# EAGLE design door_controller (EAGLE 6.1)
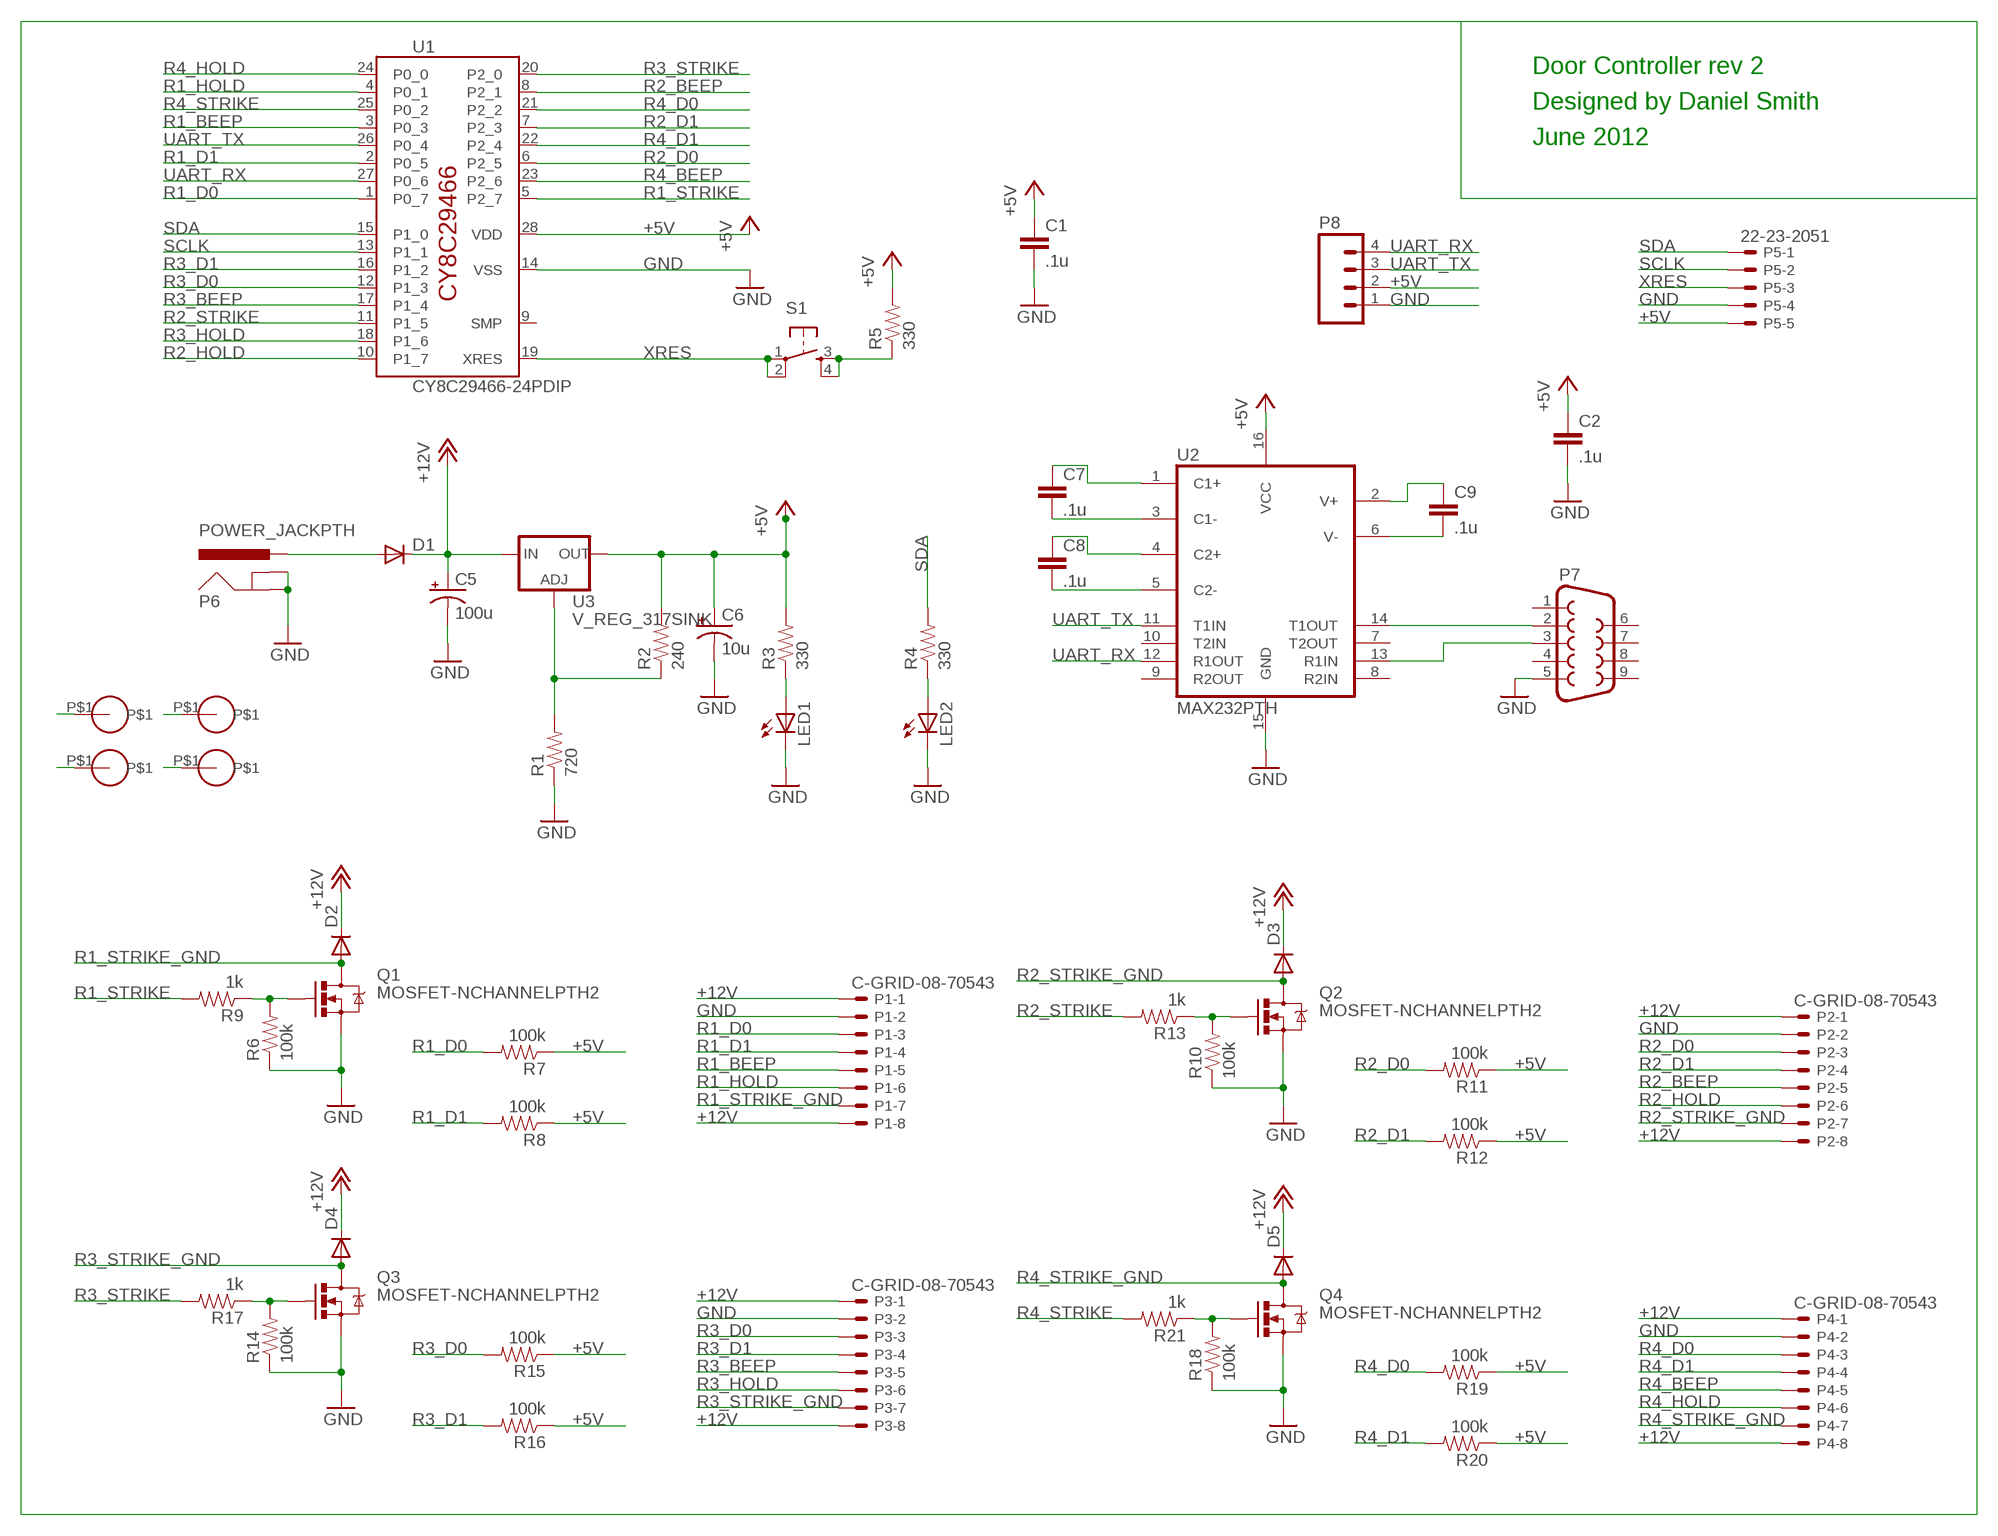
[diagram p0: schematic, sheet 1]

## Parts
C1  .1u  CAPPTH1  [CAP-PTH-5MM]
C2  .1u  CAPPTH1  [CAP-PTH-5MM]
C5  100u  CAP_POLPTH1  [CPOL-RADIAL-100UF-25V]
C6  10u  CAP_POLPTH2  [CPOL-RADIAL-10UF-25V]
C7  .1u  CAPPTH1  [CAP-PTH-5MM]
C8  .1u  CAPPTH1  [CAP-PTH-5MM]
C9  .1u  CAPPTH1  [CAP-PTH-5MM]
D1  DIODE1N4148  [DIODE-1N4148]
D2  DIODEPTH  [DIODE-1N4001]
D3  DIODEPTH  [DIODE-1N4001]
D4  DIODEPTH  [DIODE-1N4001]
D5  DIODEPTH  [DIODE-1N4001]
LED1  LED3MM  [LED3MM]
LED2  LED3MM  [LED3MM]
P1  C-GRID-08-70543  [70543-08]
P2  C-GRID-08-70543  [70543-08]
P3  C-GRID-08-70543  [70543-08]
P4  C-GRID-08-70543  [70543-08]
P5  22-23-2051  [22-23-2051]
P6  POWER_JACKPTH  [POWER_JACK_PTH]
P7  DB9FEMALE  [DB9]
P8  M04LONGPADS  [1X04_LONGPADS]
Q1  MOSFET-NCHANNELPTH2  [TO220V]
Q2  MOSFET-NCHANNELPTH2  [TO220V]
Q3  MOSFET-NCHANNELPTH2  [TO220V]
Q4  MOSFET-NCHANNELPTH2  [TO220V]
R1  720  RESISTORAXIAL-0.3  [AXIAL-0.3]
R2  240  RESISTORAXIAL-0.3  [AXIAL-0.3]
R3  330  RESISTORAXIAL-0.3  [AXIAL-0.3]
R4  330  RESISTORAXIAL-0.3  [AXIAL-0.3]
R5  330  RESISTORAXIAL-0.3  [AXIAL-0.3]
R6  100k  RESISTORAXIAL-0.3  [AXIAL-0.3]
R7  100k  RESISTORAXIAL-0.3  [AXIAL-0.3]
R8  100k  RESISTORAXIAL-0.3  [AXIAL-0.3]
R9  1k  RESISTORAXIAL-0.3  [AXIAL-0.3]
R10  100k  RESISTORAXIAL-0.3  [AXIAL-0.3]
R11  100k  RESISTORAXIAL-0.3  [AXIAL-0.3]
R12  100k  RESISTORAXIAL-0.3  [AXIAL-0.3]
R13  1k  RESISTORAXIAL-0.3  [AXIAL-0.3]
R14  100k  RESISTORAXIAL-0.3  [AXIAL-0.3]
R15  100k  RESISTORAXIAL-0.3  [AXIAL-0.3]
R16  100k  RESISTORAXIAL-0.3  [AXIAL-0.3]
R17  1k  RESISTORAXIAL-0.3  [AXIAL-0.3]
R18  100k  RESISTORAXIAL-0.3  [AXIAL-0.3]
R19  100k  RESISTORAXIAL-0.3  [AXIAL-0.3]
R20  100k  RESISTORAXIAL-0.3  [AXIAL-0.3]
R21  1k  RESISTORAXIAL-0.3  [AXIAL-0.3]
S1  TAC_SWITCHPTH  [TACTILE-PTH]
U1  CY8C29466-24PDIP  [PDIP28]
U2  MAX232PTH  [DIL16]
U3  V_REG_317SINK  [TO220-ADJ]
U$1  GNDHOLE  [GNDHOLE]
U$2  GNDHOLE  [GNDHOLE]
U$3  GNDHOLE  [GNDHOLE]
U$4  GNDHOLE  [GNDHOLE]

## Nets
+5V: C1.1 C2.1 C6.1(+) P5.5 P8.2 R2.P$2 R3.P$2 R5.P$2 R7.P$1 R8.P$1 R11.P$1 R12.P$1 R15.P$1 R16.P$1 R19.P$1 R20.P$1 U1.28(VDD) U2.16(VCC) U3.OUT
+12V [power]: C5.1(+) D1.C D2.C D3.C D4.C D5.C P1.1 P1.8 P2.1 P2.8 P3.1 P3.8 P4.1 P4.8 U3.IN
GND: C1.2 C2.2 C5.2(-) C6.2(-) LED1.K(C) LED2.K(C) P1.2 P2.2 P3.2 P4.2 P5.4 P6.GND P6.GNDBREAK P7.5 P8.1 Q1.3(S) Q2.3(S) Q3.3(S) Q4.3(S) R1.P$1 R6.P$1 R10.P$1 R14.P$1 R18.P$1 U1.14(VSS) U2.15(GND)
N$1: C7.1 U2.1(C1+)
N$2: C7.2 U2.3(C1-)
N$3: C8.1 U2.4(C2+)
N$4: C8.2 U2.5(C2-)
N$5: C9.1 U2.2(V+)
N$6: C9.2 U2.6(V-)
N$7: P7.2 U2.14(T1OUT)
N$8: P7.3 U2.13(R1IN)
N$9: U$4.P$1
N$10: R1.P$2 R2.P$1 U3.ADJ
N$11: R5.P$1 S1.3 S1.4
N$12: LED1.A R3.P$1
N$13: U$3.P$1
N$14: Q1.1(G) R6.P$2 R9.P$1
N$15: Q2.1(G) R10.P$2 R13.P$1
N$16: Q3.1(G) R14.P$2 R17.P$1
N$17: Q4.1(G) R18.P$2 R21.P$1
N$18: U$2.P$1
N$19: U$1.P$1
N$20: LED2.A R4.P$1
PWR_IN [power]: D1.A P6.PWR
R1_BEEP: P1.5 U1.3(P0_3)
R1_D0: P1.3 R7.P$2 U1.1(P0_7)
R1_D1: P1.4 R8.P$2 U1.2(P0_5)
R1_HOLD: P1.6 U1.4(P0_1)
R1_STRIKE: R9.P$2 U1.5(P2_7)
R1_STRIKE_GND [power]: D2.A P1.7 Q1.2(D)
R2_BEEP: P2.5 U1.8(P2_1)
R2_D0: P2.3 R11.P$2 U1.6(P2_5)
R2_D1: P2.4 R12.P$2 U1.7(P2_3)
R2_HOLD: P2.6 U1.10(P1_7)
R2_STRIKE: R13.P$2 U1.11(P1_5)
R2_STRIKE_GND [power]: D3.A P2.7 Q2.2(D)
R3_BEEP: P3.5 U1.17(P1_4)
R3_D0: P3.3 R15.P$2 U1.12(P1_3)
R3_D1: P3.4 R16.P$2 U1.16(P1_2)
R3_HOLD: P3.6 U1.18(P1_6)
R3_STRIKE: R17.P$2 U1.20(P2_0)
R3_STRIKE_GND [power]: D4.A P3.7 Q3.2(D)
R4_BEEP: P4.5 U1.23(P2_6)
R4_D0: P4.3 R19.P$2 U1.21(P2_2)
R4_D1: P4.4 R20.P$2 U1.22(P2_4)
R4_HOLD: P4.6 U1.24(P0_0)
R4_STRIKE: R21.P$2 U1.25(P0_2)
R4_STRIKE_GND [power]: D5.A P4.7 Q4.2(D)
SCLK: P5.2 U1.13(P1_1)
SDA: P5.1 R4.P$2 U1.15(P1_0)
UART_RX: P8.4 U1.27(P0_6) U2.12(R1OUT)
UART_TX: P8.3 U1.26(P0_4) U2.11(T1IN)
XRES: P5.3 S1.1 S1.2 U1.19(XRES)
Unconnected: P7.1 P7.4 P7.6 P7.7 P7.8 P7.9 U1.9(SMP) U2.7(T2OUT) U2.8(R2IN) U2.9(R2OUT) U2.10(T2IN)

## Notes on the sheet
- Door Controller rev 2
- Designed by Daniel Smith
- June 2012

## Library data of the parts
C1 C2 C7-C9 = SparkFun-Passives:CAP: Capacitor
C5 C6 = SparkFun-Passives:CAP_POL: Capacitor Polarized
D1-D5 = SparkFun-DiscreteSemi:DIODE: Diode
LED1 LED2 = SparkFun-LED:LED: LEDs
P1-P4 = con-molex:C-GRID-08: CONNECTOR wire to board 2.54 mm (0.100") pitch header; OC_FARNELL: unknown; OC_NEWARK: unknown
P5 = con-molex:22-23-2051: .100" (2.54mm) Center Header - 5 Pin; MF: MOLEX; MPN: 22-23-2051; OC_FARNELL: 1462952; OC_NEWARK: 38C9178
P6 = SparkFun-Connectors:POWER_JACK: Power Jack This is the standard 5.5mm barrel jack for power. The PTH is the most common, proven, reliable, footprint. All others are experimental. The Slot footprint only works if the mill layer is transmitted to the PCB fab house so be warned. Spark Fun Electronics SKU : PRT-00119. Mating wall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
P7 = SparkFun-Connectors:DB9: DB9 Connector Standard DB9 (D-Sub 9) serial connector. Can be used for CAN bus as well as RS485 and RS232. Footprint production proven. Spark Fun Electronics SKU : PRT-00429
P8 = SparkFun-Connectors:M04: Header 4 Standard 4-pin 0.1" header. Use with straight break away headers (SKU : PRT-00116), right angle break away headers (PRT-00553), swiss pins (PRT-00743), machine pins (PRT-00117), and female headers (PRT-00115). Molex polarized connector foot print use with SKU : PRT-08231 with associated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
Q1-Q4 = SparkFun-DiscreteSemi:MOSFET-NCHANNEL: Generic NMOS footprint
R1-R21 = SparkFun-Passives:RESISTOR: Resistor
S1 = SparkFun-Electromechanical:TAC_SWITCH: Momentary Switch Button commonly used for reset or general input. Spark Fun Electronics SKU : COM-00097
U1 = cypress-psoc:CY8C29466-24*
U2 = SparkFun-DigitalIC:MAX232: RS232 Transceiver Very common IC. This is generically called 'MAX232', but works with the 3V equivalent MAX3232 generic ICs. Field tested and mother approved. Spark Fun Electronics SKU : COM-00316 (DIP) and COM-00589 (SMD)
U3 = SparkFun-PowerIC:V_REG_317: Voltage Regulator Standard LM317 adjustable voltage regulator. AOI (Adjust Output Input). Google 'LM317 Calculator' for easy to use app to get the two resistor values needed. 240/720 for 5V output. 240/390 for 3.3V output. Spark Fun Electronics SKU : COM-00527
U$1-U$4 = GT-IEEE:GNDHOLE

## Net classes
0 default: clearance 0.508 mm
1 power: width 0.508 mm, clearance 0.508 mm

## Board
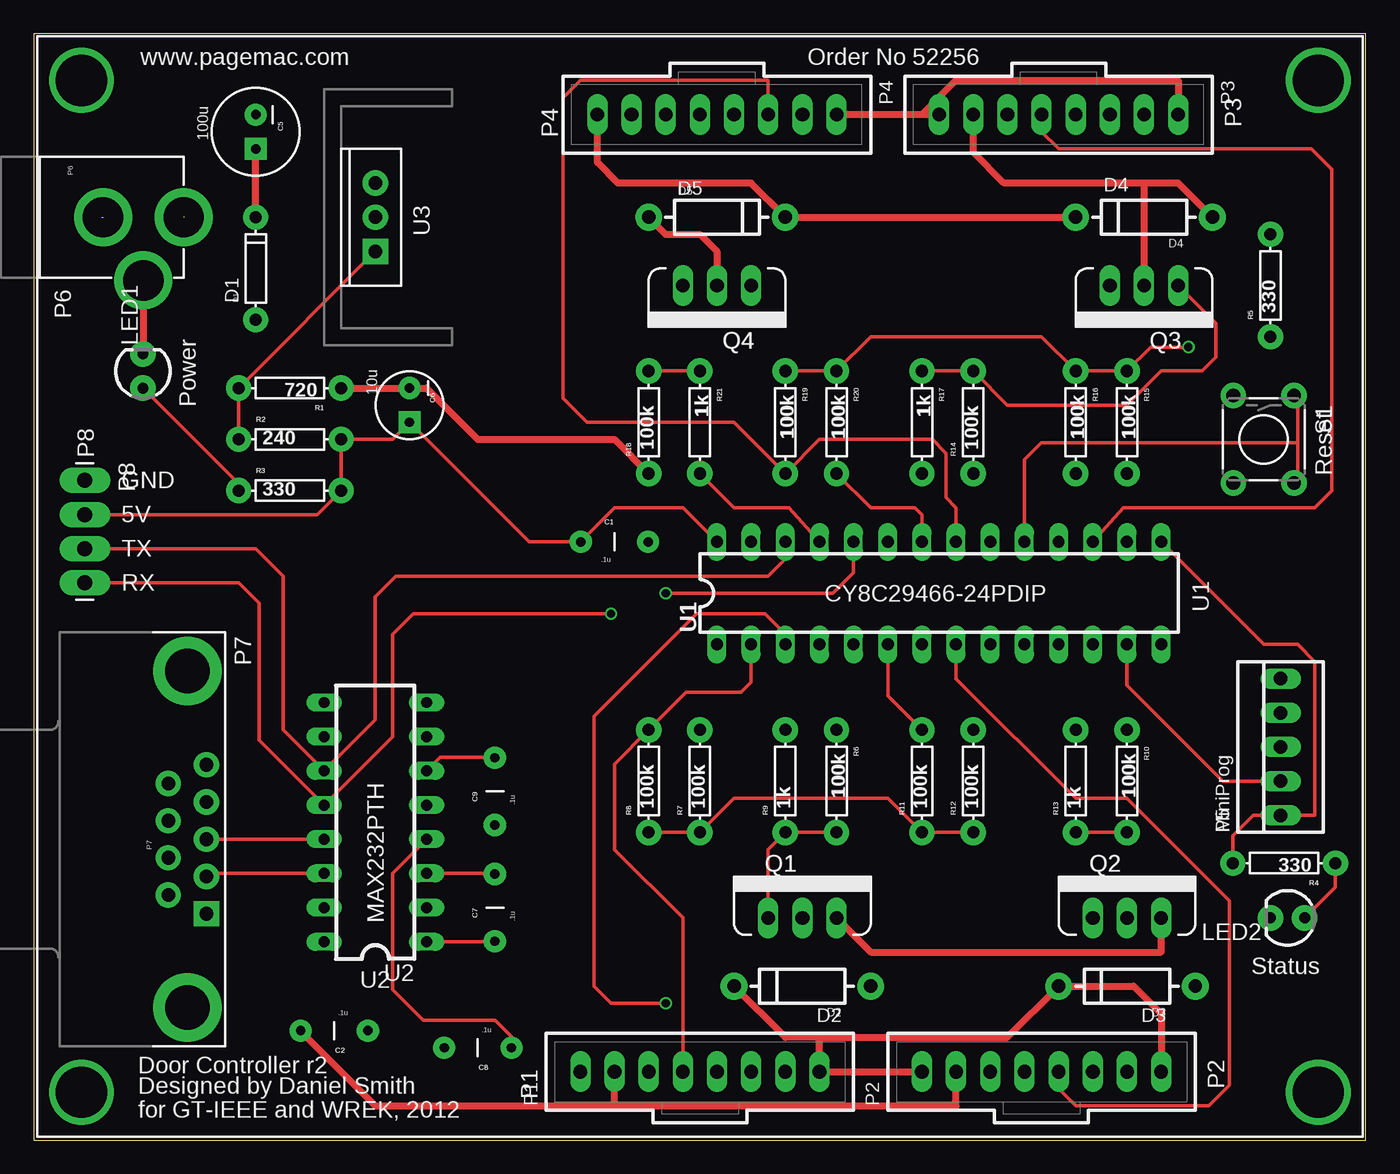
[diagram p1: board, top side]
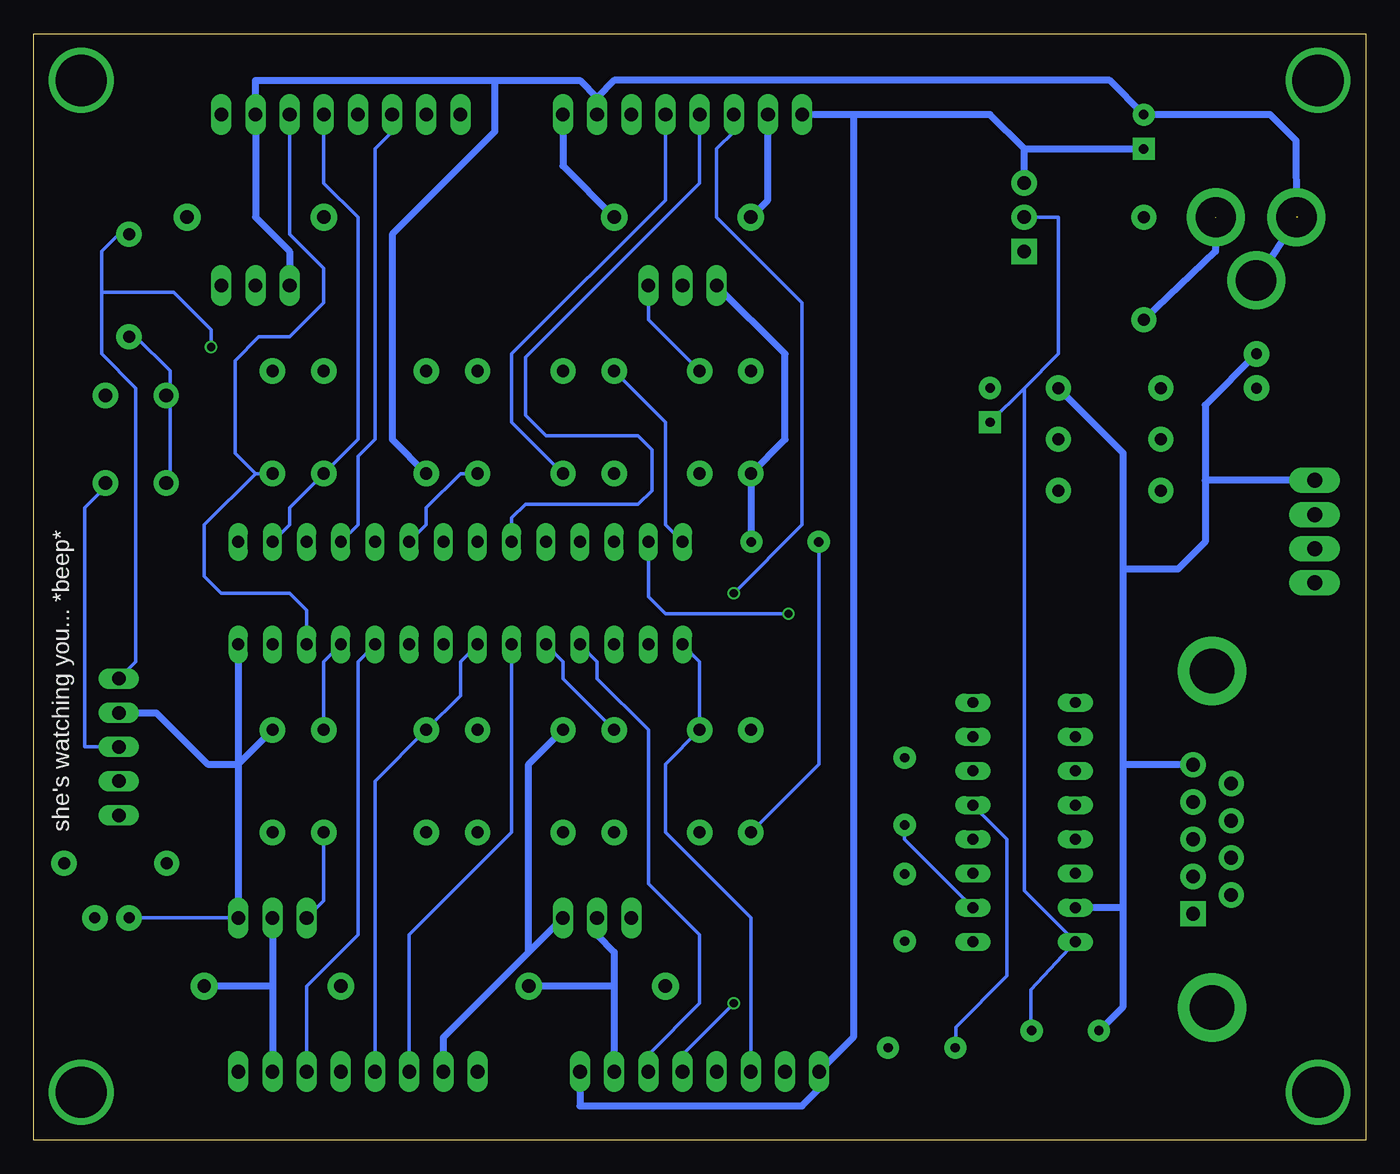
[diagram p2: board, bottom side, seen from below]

Size 99.04 x 82.22 mm. Coordinates in mm from the lower left corner, seen from the top.
Outline: 0,0 99.04,0 99.04,82.22 0,82.22 0,0
Copper layers (1*16): Top 0.035mm / dielectric 1.5mm / Bottom 0.035mm
Design rules: minimum track width 6mil, minimum drill 12mil, track to track 6mil, track to pad 6mil, pad to pad 6mil, via to via 6mil, smd to smd 0mil, copper to edge 10mil, drill to drill 10mil, minimum pad ring 10mil, minimum via ring 6mil, stop-mask expansion 2mil, vias tented up to drill 100mil, thermal gap 10mil

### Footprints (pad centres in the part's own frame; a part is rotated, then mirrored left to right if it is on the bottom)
CAP-PTH-5MM = drill 0.7 pad 1.651: 1 -2.5,0; 2 2.5,0
CPOL-RADIAL-100UF-25V = drill 0.7 pad 1.651 square: 1 1.27,0 | drill 0.7 pad 1.651: 2 -1.27,0
CPOL-RADIAL-10UF-25V = drill 0.7 pad 1.651 square: 1 1.27,0 | drill 0.7 pad 1.651: 2 -1.27,0
DIODE-1N4148 = drill 0.9 pad 1.88: A -3.81,0; C 3.81,0
DIODE-1N4001 = drill 1 pad 1.981: A -5.08,0; C 5.08,0
LED3MM = drill 0.813 pad 1.88: A -1.27,0; K 1.27,0
70543-08 = drill 1.016 long: 1 -8.89,0; 2 -6.35,0; 3 -3.81,0; 4 -1.27,0; 5 1.27,0; 6 3.81,0; 7 6.35,0; 8 8.89,0
22-23-2051 = drill 1 long: 1 -5.08,0; 2 -2.54,0; 3 0,0; 4 2.54,0; 5 5.08,0
POWER_JACK_PTH = drill 2.997 pad 4.318: GND 0,7.7; GNDBREAK 4.7,10.7; PWR 0,13.7
DB9 = drill 1.016 pad 1.88 square: 1 -5.54,-1.42 | drill 1.016 pad 1.88: 2 -2.77,-1.42; 3 0,-1.42; 4 2.77,-1.42; 5 5.54,-1.42; 6 -4.15,1.42; 7 -1.38,1.42; 8 1.38,1.42; 9 4.15,1.42 | drill 3.302 pad 5.08: G1 -12.5,0; G2 12.5,0
1X04_LONGPADS = drill 1.118 pad 1.88 long: 1 0,0; 2 2.54,0; 3 5.08,0; 4 7.62,0
TO220V = drill 1.016 long: 1 -2.54,0; 2 0,0; 3 2.54,0
AXIAL-0.3 = drill 0.9 pad 1.88: P$1 -3.81,0; P$2 3.81,0
TACTILE-PTH = drill 1.016 pad 1.88: 1 -3.251,2.261; 2 3.251,2.261; 3 -3.251,-2.261; 4 3.251,-2.261
PDIP28 = drill 0.889 long: 1 -16.51,-3.81; 2 -13.97,-3.81; 3 -11.43,-3.81; 4 -8.89,-3.81; 5 -6.35,-3.81; 6 -3.81,-3.81; 7 -1.27,-3.81; 8 1.27,-3.81; 9 3.81,-3.81; 10 6.35,-3.81; 11 8.89,-3.81; 12 11.43,-3.81; 13 13.97,-3.81; 14 16.51,-3.81; 15 16.51,3.81; 16 13.97,3.81; 17 11.43,3.81; 18 8.89,3.81; 19 6.35,3.81; 20 3.81,3.81; 21 1.27,3.81; 22 -1.27,3.81; 23 -3.81,3.81; 24 -6.35,3.81; 25 -8.89,3.81; 26 -11.43,3.81; 27 -13.97,3.81; 28 -16.51,3.81
DIL16 = drill 0.813 long: 1 -8.89,-3.81; 2 -6.35,-3.81; 3 -3.81,-3.81; 4 -1.27,-3.81; 5 1.27,-3.81; 6 3.81,-3.81; 7 6.35,-3.81; 8 8.89,-3.81; 9 8.89,3.81; 10 6.35,3.81; 11 3.81,3.81; 12 1.27,3.81; 13 -1.27,3.81; 14 -3.81,3.81; 15 -6.35,3.81; 16 -8.89,3.81
TO220-ADJ = drill 1 pad 1.88 square: ADJ -2.54,0 | drill 1 pad 1.88: IN 2.54,0; OUT 0,0
GNDHOLE = drill 3.81: P$1 0,0

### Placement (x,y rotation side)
C1  43.18,44.45 0 top
C2  22.35,8.13 180 top
C5  16.51,74.93 270 top
C6  27.94,54.61 270 top
C7  34.29,17.27 90 top
C8  33.02,6.86 180 top
C9  34.29,25.91 90 top
D1  16.51,64.77 90 top
D2  57.15,11.43 180 top
D3  81.28,11.43 180 top
D4  82.55,68.58 180 top
D5  50.8,68.58 0 top
LED1  8.13,57.15 90 top
LED2  93.22,16.51 180 top
P1  49.53,5.08 0 top
P2  74.93,5.08 0 top
P3  76.2,76.2 180 top
P4  50.8,76.2 180 top
P5  92.71,29.21 90 top
P6  -2.54,68.58 270 top
P7  11.43,22.35 90 top
P8  3.81,49.02 270 top
Q1  57.15,16.51 0 top
Q2  81.28,16.51 0 top
Q3  82.55,63.5 180 top
Q4  50.8,63.5 180 top
R1  19.05,55.88 180 top
R2  19.05,52.07 0 top
R3  19.05,48.26 0 top
R4  92.96,20.57 180 top
R5  91.95,63.5 90 top
R6  59.69,26.67 270 top
R7  49.53,26.67 90 top
R8  45.72,26.67 90 top
R9  55.88,26.67 90 top
R10  81.28,26.67 270 top
R11  66.04,26.67 90 top
R12  69.85,26.67 90 top
R13  77.47,26.67 90 top
R14  69.85,53.34 90 top
R15  81.28,53.34 270 top
R16  77.47,53.34 270 top
R17  66.04,53.34 270 top
R18  45.72,53.34 90 top
R19  55.88,53.34 270 top
R20  59.69,53.34 270 top
R21  49.53,53.34 270 top
S1  91.44,52.07 270 top
U1  67.31,40.64 0 top
U2  25.4,23.62 90 top
U3  25.4,68.58 90 top
U$1  3.56,3.56 0 top
U$2  95.5,3.56 0 top
U$3  3.56,78.74 0 top
U$4  95.5,78.74 0 top

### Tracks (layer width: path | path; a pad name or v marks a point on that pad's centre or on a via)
+5V  (via drill 0.61)
  Top 0.254: R12.P$1 R11.P$1 63.5,25.4 52.07,25.4 R7.P$1 R8.P$1 | R19.P$1 R20.P$1 62.23,59.69 74.93,59.69 R16.P$1 R15.P$1 83.06,58.93 v85.85,58.93 | U1.28 48.26,46.99 43.18,46.99 40.64,44.45 | 40.64,44.45 36.83,44.45 C6.1 26.67,52.07 R2.P$2 R3.P$2 21.08,46.48 P8.2 | 40.64,44.45 C1.1
  Bottom 0.254: C2.1 24.89,8.13 24.89,11.18 U2.16 25.4,18.54 25.4,55.88 | U3.OUT 22.86,68.58 22.86,58.42 25.4,55.88 | C6.1 25.4,55.88 | P5.5 91.44,35.56 91.44,55.88 93.98,58.42 93.98,62.99 | 93.98,62.99 93.98,66.04 92.71,67.31 R5.P$2 | R8.P$1 40.64,27.94 40.64,44.45 C1.1 | R19.P$1 52.07,53.34 52.07,45.72 U1.28 | v85.85,58.93 85.85,60.2 88.65,62.99 93.98,62.99
+12V
  Top 0.508: P2.1 P1.8 58.42,7.62 | D2.C 55.88,7.62 58.42,7.62 | 58.42,7.62 72.39,7.62 D3.C 81.79,11.43 83.82,9.4 P2.8 | D1.C C5.1 | P3.8 66.04,76.2 | 66.04,76.2 P4.1 | P3.1 85.09,78.74 68.58,78.74 66.04,76.2 | D4.C D5.C 53.34,71.12 43.43,71.12 41.91,72.64 P4.8
  Bottom 0.508: P1.8 58.42,2.54 41.91,2.54 40.64,3.81 P1.1 38.1,7.62 38.1,76.2 | 38.1,76.2 27.94,76.2 25.4,73.66 | 38.1,76.2 P4.8 | U3.IN 25.4,73.66 | 25.4,73.66 C5.1 | D5.C 59.69,72.39 P4.1
GND  (1 unrouted)
  Top 0.508: LED1.K 8.13,63.75 P6.GNDBREAK | R1.P$1 C6.2 29.21,55.88 33.02,52.07 43.18,52.07 R18.P$1 | 43.18,2.54 P1.2 | 43.18,2.54 25.4,2.54 20.07,7.87 C2.2 | P2.2 68.58,2.54 43.18,2.54 | Q2.3 83.82,13.97 62.23,13.97 Q1.3
  Bottom 0.254: LED2.K Q2.3
  Bottom 0.508: U1.14 83.82,27.94 | LED1.K 11.94,54.61 11.94,49.02 | 11.94,49.02 11.94,44.45 13.97,42.42 18.03,42.42 | 57.15,77.47 58.42,78.74 64.77,78.74 | 64.77,78.74 82.55,78.74 P3.2 82.55,68.58 80.01,66.04 Q3.3 | R14.P$1 72.39,52.07 72.39,67.31 64.77,74.93 64.77,78.74 | 5.08,68.58 P6.GNDBREAK | P6.GND 5.21,74.3 7.11,76.2 C5.2 19.05,78.74 55.88,78.74 57.15,77.47 | 83.82,27.94 Q2.3 | 83.82,27.94 R10.P$1 | Q4.3 43.18,58.42 43.18,52.07 R18.P$1 45.72,44.45 C1.2 | 18.03,17.27 U2.15 | 18.03,17.27 18.03,9.91 19.81,8.13 C2.2 | 62.23,13.97 68.58,7.62 P2.2 | 62.23,13.97 Q1.3 | 18.03,27.94 12.7,27.94 P7.5 | 18.03,17.27 18.03,27.94 | R6.P$1 62.23,27.94 62.23,13.97 | R1.P$1 18.03,51.05 18.03,42.42 | 18.03,27.94 18.03,42.42 | 57.15,77.47 P4.2 | P5.4 89.92,31.75 86.11,27.94 83.82,27.94 | P8.1 11.94,49.02
N$1
  Top 0.254: U2.1 34.29,14.73 C7.1
N$2
  Top 0.254: U2.3 34.29,19.81 C7.2
N$3
  Top 0.254: U2.4 26.67,19.81 26.67,11.18 28.96,8.89 34.29,8.89 35.56,7.62 C8.1
N$4
  Bottom 0.254: U2.5 26.67,22.35 26.67,12.19 30.48,8.38 C8.2
N$5
  Bottom 0.254: U2.2 34.29,22.35 C9.1
N$6
  Top 0.254: U2.6 30.23,28.45 34.29,28.45 C9.2
N$7
  Top 0.254: U2.14 12.7,19.81 P7.2
N$8
  Top 0.254: U2.13 P7.3 12.7,22.35
N$10
  Top 0.254: R2.P$1 R1.P$2 U3.ADJ
N$11
  Bottom 0.254: S1.4 88.9,49.53 88.9,54.61 S1.3 88.9,55.88 88.9,57.15 91.44,59.69 R5.P$1
N$12
  Top 0.254: LED1.A 15.24,48.77 R3.P$1
N$14
  Top 0.254: Q1.1 54.61,21.59 R9.P$1 R6.P$2
N$15
  Top 0.254: R13.P$1 R10.P$2
  Bottom 0.254: Q2.1 77.47,17.78 R13.P$1
N$16
  Top 0.254: Q3.1 87.88,60.71 87.88,58.17 86.87,57.15 83.82,57.15 81.28,54.61 72.39,54.61 R14.P$2 R17.P$1
N$17
  Top 0.254: R21.P$1 R18.P$2
  Bottom 0.254: Q4.1 53.34,60.96 R21.P$1
N$20
  Top 0.254: R4.P$1 96.77,18.8 LED2.A
PWR_IN  (1 unrouted)
  Bottom 0.508: D1.A 11.18,66.04 11.18,68.58
R1_BEEP  (via drill 0.61)
  Top 0.254: v46.99,10.16 42.93,10.16 41.66,11.43 41.66,31.5 49.28,39.12 54.36,39.12 55.63,37.85 U1.3
  Bottom 0.254: v46.99,10.16 50.8,6.35 P1.5
R1_D0
  Bottom 0.254: U1.1 49.53,35.56 R7.P$2 52.07,27.94 52.07,22.86 45.72,16.51 P1.3
R1_D1
  Top 0.254: P1.4 48.26,16.51 43.18,21.59 43.18,27.94 R8.P$2 48.51,33.27 52.58,33.27 53.34,34.04 U1.2
R1_HOLD
  Bottom 0.254: U1.4 57.15,35.56 57.15,34.29 53.34,30.48 53.34,19.05 49.53,15.24 49.53,10.16 53.34,6.35 P1.6
R1_STRIKE
  Bottom 0.254: U1.5 59.69,35.56 59.69,34.29 R9.P$2
R1_STRIKE_GND
  Bottom 0.508: 55.88,11.43 55.88,13.97 57.15,15.24 Q1.2 | 55.88,11.43 P1.7 | 55.88,11.43 D2.A
R2_BEEP
  Top 0.254: P2.5 76.2,3.81 77.47,2.54 87.38,2.54 88.9,4.06 88.9,17.78 81.28,25.4 80.26,25.4 80.01,25.4 77.47,25.4 68.58,34.29 U1.8
R2_D0
  Top 0.254: U1.6 63.5,33.02 R11.P$2
  Bottom 0.254: P2.3 71.12,15.24 63.5,22.86 U1.6
R2_D1
  Bottom 0.254: U1.7 67.31,35.56 67.31,33.02 R12.P$2 73.66,26.67 P2.4
R2_HOLD
  Bottom 0.254: U1.10 74.93,35.56 74.93,15.24 78.74,11.43 P2.6
R2_STRIKE
  Bottom 0.254: U1.11 77.47,35.56 R13.P$2
R2_STRIKE_GND
  Bottom 0.508: Q2.2 81.28,11.43 | 81.28,11.43 P2.7 | 81.28,11.43 D3.A
R3_BEEP
  Top 0.254: U1.17 81.03,46.99 95.25,46.99 96.52,48.26 96.52,72.14 95,73.66 76.2,73.66 74.93,74.93 P3.5
R3_D0
  Bottom 0.254: U1.12 78.74,39.37 80.01,40.64 85.09,40.64 86.36,41.91 86.36,45.72 82.55,49.53 | R15.P$2 82.55,49.53 | P3.3 80.01,67.31 77.47,64.77 77.47,62.23 80.01,59.69 82.3,59.69 84.07,57.91 84.07,51.05 82.55,49.53
R3_D1
  Bottom 0.254: U1.16 80.01,45.72 80.01,46.99 R16.P$2 74.93,52.07 74.93,68.58 77.47,71.12 P3.4
R3_HOLD
  Bottom 0.254: U1.18 74.93,45.72 74.93,50.8 73.66,52.07 73.66,73.66 72.39,74.93 P3.6
R3_STRIKE
  Bottom 0.254: U1.20 69.85,45.72 69.85,46.99 67.31,49.53 R17.P$2
R3_STRIKE_GND
  Top 0.508: P3.7 69.85,73.41 72.14,71.12 82.55,71.12 | 82.55,71.12 85.09,71.12 D4.A | 82.55,71.12 Q3.2
R4_BEEP
  Bottom 0.254: P4.5 49.53,71.12 62.48,58.17 62.48,53.85 60.96,52.32 54.1,52.32 53.09,51.31 53.09,48.26 54.1,47.24 62.48,47.24 63.5,46.23 U1.23
R4_D0
  Top 0.254: U1.21 68.58,46.99 67.82,47.75 67.82,51.05 66.8,52.07 58.42,52.07 R19.P$2 52.07,53.34 41.15,53.34 39.37,55.12 39.37,77.47 40.64,78.74 54.61,78.74 P4.3
R4_D1
  Top 0.254: R20.P$2 62.23,46.99 65.53,46.99 66.04,46.48 U1.22
  Bottom 0.254: P4.4 52.07,69.85 63.5,58.42 63.5,53.34 R20.P$2
R4_HOLD  (via drill 0.61)
  Top 0.254: v46.99,40.64 59.44,40.64 60.96,42.16 U1.24
  Bottom 0.254: v46.99,40.64 41.91,45.72 41.91,62.23 48.26,68.58 48.26,73.66 46.99,74.93 P4.6
R4_STRIKE
  Top 0.254: U1.25 56.13,46.99 52.07,46.99 R21.P$2
R4_STRIKE_GND
  Top 0.508: D5.A 46.99,67.31 49.53,67.31 50.8,66.04 Q4.2
  Bottom 0.508: P4.7 44.45,69.85 D5.A
SCLK
  Top 0.254: U1.13 81.28,33.78 88.39,26.67 P5.2
SDA
  Top 0.254: U1.15 91.44,36.83 93.98,36.83 95.25,35.56 95.25,24.13 P5.1 90.68,24.13 89.15,22.61 R4.P$2
UART_RX  (via drill 0.61)
  Top 0.254: v42.93,39.12 28.19,39.12 26.67,37.59 26.67,29.97 U2.12 16.76,29.72 16.76,39.88 15.24,41.4 P8.4
  Bottom 0.254: U1.27 53.34,40.39 52.07,39.12 v42.93,39.12
UART_TX
  Top 0.254: U1.26 55.88,43.18 54.61,41.91 26.92,41.91 25.4,40.39 25.4,31.24 U2.11 18.54,30.48 18.54,41.91 16.51,43.94 P8.3
XRES
  Top 0.254: S1.2 93.98,49.53 93.98,51.82 | 93.98,51.82 93.98,54.61 S1.1 | U1.19 73.66,50.55 74.93,51.82 93.98,51.82
  Bottom 0.254: P5.3 95.25,29.21 95.25,46.99 93.98,48.26 S1.2

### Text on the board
_tsilk: www.pagemac.com | Order No 52256 | 100u | P4 | P3 | C5 | D4 | D5 | U3 | P6 | D1 | R5 | 330 | Q4 | Q3 | 10u | 720 | R21 | R19 | R20 | R17 | R16 | R15 | R1 | C6 | 1k | 100k | 100k | 1k | 100k | 100k | Power | Reset | P8 | R2 | 240 | R18 | 100k | R14 | 100k | R3 | GND | 330 | 5V | C1 | TX | .1u | RX | CY8C29466-24PDIP | U1 | P7 | 100k | R6 | 100k | R10 | C9 | .1u | 100k | 100k | 1k | 100k | 100k | 1k | R8 | R7 | R9 | R11 | R12 | R13 | MiniProg | 330 | Q1 | Q2 | R4 | C7 | MAX232PTH | .1u | Status | U2 | .1u | D2 | D3 | .1u | C2 | Door Controller r2 | C8 | Designed by Daniel Smith | P2 | for GT-IEEE and WREK, 2012 | P1
_bsilk: she's watching you... *beep*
